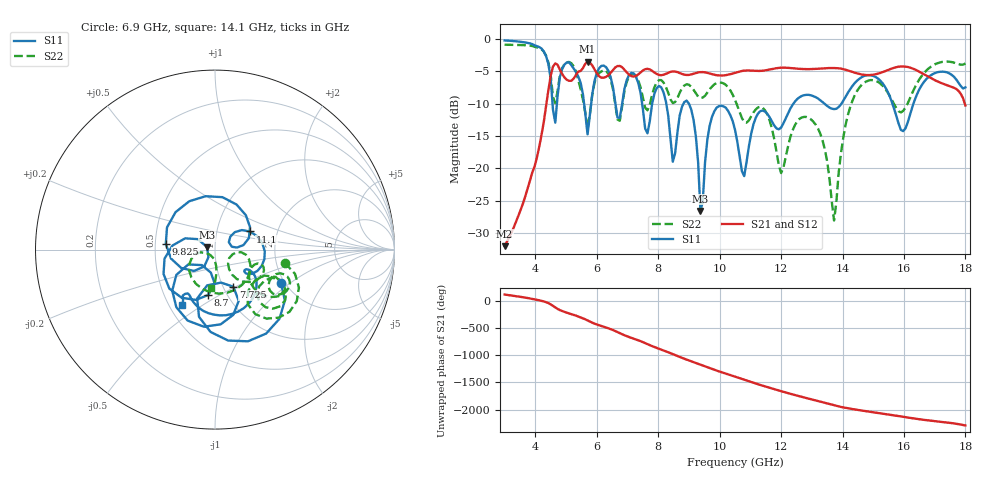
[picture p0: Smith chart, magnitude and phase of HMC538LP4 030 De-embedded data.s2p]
! Chelmsford, MA 01824
! http://www.hittite.com
! Tel: 978-250-3343
! Fax: 978-250-3373
! Device  :  HMC538LP4
! Description:  600 Analog Phase Shifter
! Frequency  :  6.0 GHz - 15.0 GHz
! Package  :  LP4  - 4x4 mm Quad Flatpack No-Lead (QFN) Plastic Package: 24 pin
! Ports  :  2 RF, 1 DC
!  Pin  3  = Rfin  = Port 1
!  Pin  16  = Rfout = Port 2
!  pin  21  = vCTL
! Voltages:  VCTL  = 0 to 5.0 Volts
! Currents :  Vb(V)  Vd(V)  Ib(mA)  Id(mA)
!  0.00  3.00  0.000000	0.472387
! Data:  The device was measured on evaluation board 111296-1.
!  Data was collected using a calibrated network analyzer.
!  The evaluation circuit board was modeled and simulated.This was use
!  to removed the evaluation board circuit from the measured data.
!  The reference plane is the center of the package pin.
! Misc:  Lot #
!Date Measured:  03 - 11 -2009
! Date:  03 - 17 -2009
! Note:
!  Hittite Microwave supplies this data as a sample of measured data at the
!  package pin for this package product.  Your particular data for this product
!  may vary.
!  Data was taken at 25 degrees C.
!  Hittite Microwave reserves the right to change this data at anytime.
# MHz S MA R 50
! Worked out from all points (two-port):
!   201 points, 3 GHz to 18 GHz, reference 50 ohm
!   highest |S21| = -3.48 dB at 5.7 GHz (marker M1); lowest = -32.0 dB at 3 GHz (marker M2)
!   |S21| within 3 dB of the highest: 4.473 GHz to 17.06 GHz (12.59 GHz wide, 117 % of centre)
!   lowest |S11| = -26.6 dB at 9.375 GHz (marker M3), VSWR 1.10, Z = 45.7 + j1.26 ohm
!   |S11| at or under -10 dB: 9.002 GHz to 12.4 GHz (3.398 GHz wide, 31.8 % of centre); 13.42 GHz to 13.96 GHz (547.3 MHz wide, 4 % of centre); 15.62 GHz to 16.31 GHz (683.6 MHz wide, 4.28 % of centre)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
!   |S22| runs from -28.1 to -0.9 dB; largest |S21 - S12| = 0.0038
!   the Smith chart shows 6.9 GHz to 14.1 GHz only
!   S11 on the Smith chart (normalised r, x): 6.9 GHz: 1.92, -0.85; 7.725 GHz: 1.12, -0.49; 8.7 GHz: 0.82, -0.44; 9.825 GHz: 0.57, +0.04; 11.1 GHz: 1.44, +0.31; 14.1 GHz: 0.58, -0.41
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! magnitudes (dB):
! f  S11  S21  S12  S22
! 3 GHz  -0.2  -32.0  -32.1  -0.9
! 4.575 GHz  -10.9  -4.2  -4.3  -9.0
! 5.55 GHz  -8.5  -4.5  -4.5  -9.3
! 5.7 GHz  -14.7  -3.5  -3.5  -13.8
! 6.075 GHz  -4.5  -5.7  -5.7  -5.3
! 6.9 GHz  -7.7  -4.7  -4.7  -8.1
! 7.725 GHz  -12.7  -4.7  -4.7  -10.2
! 8.025 GHz  -7.2  -5.5  -5.5  -6.3
! 8.475 GHz  -19.0  -5.0  -5.0  -9.9
! 8.7 GHz  -11.8  -5.2  -5.3  -8.3
! 9.15 GHz  -12.5  -5.4  -5.4  -7.8
! 9.375 GHz  -26.6  -5.1  -5.1  -9.1
! 9.825 GHz  -11.2  -5.5  -5.5  -7.0
! 10.5 GHz  -14.0  -5.2  -5.2  -9.4
! 10.8 GHz  -21.2  -4.9  -4.9  -12.8
! 11.1 GHz  -13.2  -4.9  -4.9  -11.3
! 12 GHz  -13.7  -4.4  -4.4  -20.7
! 13.05 GHz  -8.8  -4.6  -4.6  -12.8
! 13.72 GHz  -10.8  -4.5  -4.5  -28.1
! 14.1 GHz  -8.9  -4.7  -4.8  -13.3
! 15.53 GHz  -8.7  -4.7  -4.7  -8.7
! 18 GHz  -7.5  -10.3  -10.2  -3.8
